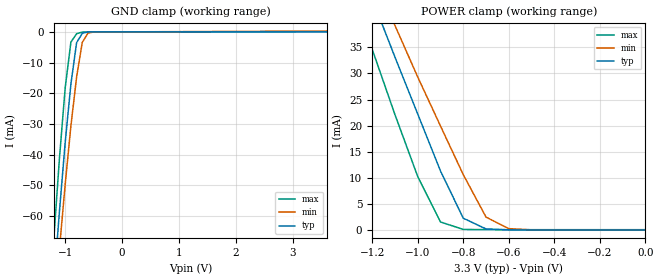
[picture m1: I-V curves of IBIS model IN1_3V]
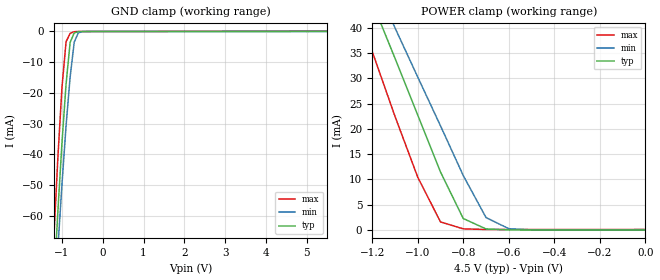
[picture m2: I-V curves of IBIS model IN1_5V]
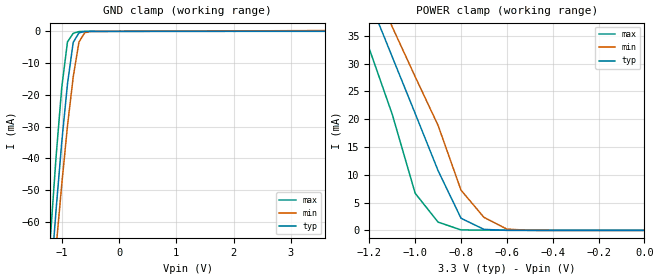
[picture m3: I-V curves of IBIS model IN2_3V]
[IBIS Ver]   5.0
[File Name]   1273na084.ibs
[File Rev]   1.0
[Date]   July 11, 2019
[Source]   JSC NIIET
[Disclaimer]
|   IBIS MODEL LICENSE AND DISCLAIMER AGREEMENT
|  Before downloading or using the below-referenced IBIS model, please read and
|  accept the license agreement and disclaimer shown below.
|   LICENSE STATEMENT
|  The information in this IBIS model is protected under the copyright laws of
|  the Russia and other countries. JSC NIIET hereby
|  grants the users of this IBIS model (hereto referred to as licensee) a
|  nonexclusive, nontransferable license to use this IBIS model as long as the
|  licensee abides by the terms of this agreement.
|  Before using the IBIS model, the licensee should read this license. By using,
|  copying, modifying or redistributing this IBIS model,licensee accepts and
|  agrees to become bound by the terms of this agreement. If the licensee does
|  not accept these terms, then the licensee should not use the IBIS model and
|  should return it to JSC NIIET immediately.
|  The licensee may not sell, loan, rent, lease, distribute or license the IBIS
|  model,in whole, in part, or in modified form, to anyone outside the
|  licensee's company. The licensee may modify the IBIS model to suit his
|  specific applications, provided that all rights in such modifications and
|  derivative works shall belong to JSC NIIET. The licensee may make copies of this
|  IBIS model for use within his company only.
|  THIS IBIS MODEL IS PROVIDED AS IS, WHERE IS, AND WITH NO WARRANTY OF ANY
|  KIND EITHER EXPRESSED OR IMPLIED, INCLUDING BUT NOT LIMITED TO ANY IMPLIED
|  WARRANTIES OF MERCHANTABILITY AND FITNESS FOR A PARTICULAR PURPOSE.
|  Licensee understands that the mathematical behavioral characteristics and
|  formulas for the IBIS model have not been fully characterized for production
|  specification or exact compliance to actual part operation. The IBIS model
|  is useful for general simulations but not intended for safety critical,
|  manufacturing yield, or similar safety or financial decision making
|  simulations. In no event will JSC NIIET be liable for indirect, special,
|  collateral, incidental, consequential or punitive damages in connection with
|  or arising out of the use of this IBIS model. JSC NIIET reserves the right to
|  make changes to its products and the IBIS model without prior notice.
|  The Parties agree that the foregoing terms constitute the entire agreement
|  and that this agreement shall be governed by and construed in accordance
|  with the laws of the Russsia, without regard to choice of law provisions.
[Copyright]
|  This model is an exclusive property of JSC NIIET
|  and is not to be resold or redistributed without the written
|  permission of JSC NIIET.
|  Copyright(c) 2019 JSC NIIET, All Rights Reserved
|   Component 1273HA084
[Component]   1273HA084
[Manufacturer] JSC NIIET
[Package]
| variable   typ   min   max
R_pkg   0   NA   NA
L_pkg   0   NA   NA
C_pkg   0   NA   NA
[Pin]   signal_name   model_name   R_pin   L_pin   C_pin
1   NC   NC   NA   NA   NA
2   #VCC   POWER   NA   NA   NA
3   NC   NC   NA   NA   NA
4   MOSI/ADR1   IN1   NA   NA   NA
5   MISO/SDA   IO   NA   NA   NA
6   SCLK/SCL   IN1   NA   NA   NA
7   SS#/ADR0   IN1   NA   NA   NA
8   SA_MODE   IN1   NA   NA   NA
9   PU/RST#   IN2   NA   NA   NA
10   NC   NC   NA   NA   NA
11   AGND   GND   NA   NA   NA
12   VCC1   POWER   NA   NA   NA
13   DAC1P   TERM   NA   NA   NA
14   DAC1N   TERM   NA   NA   NA
15   DAC2P   TERM   NA   NA   NA
16   DAC2N   TERM   NA   NA   NA
17   DAC3P   TERM   NA   NA   NA
18   DAC3N   TERM   NA   NA   NA
19   DAC4P   TERM   NA   NA   NA
20   DAC4N   TERM   NA   NA   NA
21   VCC2   POWER   NA   NA   NA
22   DAC_BIAS1   TERM   NA   NA   NA
23   DAC_BIAS2   TERM   NA   NA   NA
24   AGND   GND   NA   NA   NA
25   CM   TERM   NA   NA   NA
26   TS_REF   TERM   NA   NA   NA
27   DAC5P   TERM   NA   NA   NA
28   DAC5N   TERM   NA   NA   NA
29   DAC6P   TERM   NA   NA   NA
30   DAC6N   TERM   NA   NA   NA
31   DAC7P   TERM   NA   NA   NA
32   DAC7N   TERM   NA   NA   NA
33   DAC8P   TERM   NA   NA   NA
34   DAC8N   TERM   NA   NA   NA
35   DAC9P   TERM   NA   NA   NA
36   DAC9N   TERM   NA   NA   NA
37   DAC10P   TERM   NA   NA   NA
38   DAC10N   TERM   NA   NA   NA
39   DAC11P   TERM   NA   NA   NA
40   DAC11N   TERM   NA   NA   NA
41   DAC12P   TERM   NA   NA   NA
42   DAC12N   TERM   NA   NA   NA
43   AGND   GND   NA   NA   NA
44   DAC_BIAS3   TERM   NA   NA   NA
45   DAC_BIAS4   TERM   NA   NA   NA
46   VCC3   POWER   NA   NA   NA
47   VCC3   POWER   NA   NA   NA
48   DAC13P   TERM   NA   NA   NA
49   DAC13N   TERM   NA   NA   NA
50   DAC14P   TERM   NA   NA   NA
51   DAC14N   TERM   NA   NA   NA
52   DAC15P   TERM   NA   NA   NA
53   SUBS   TERM   NA   NA   NA
54   DAC15N   TERM   NA   NA   NA
55   VCC4   POWER   NA   NA   NA
56   AGND   GND   NA   NA   NA
57   SUBS   TERM   NA   NA   NA
58   DAC16P   TERM   NA   NA   NA
59   DAC16N   TERM   NA   NA   NA
60   PLLGND   GND   NA   NA   NA
61   LF   TERM   NA   NA   NA
62   PLLVCC   POWER   NA   NA   NA
63   MCLKI/XT1   TERM   NA   NA   NA
64   XTALO   TERM   NA   NA   NA
65   MCLKO   TERM   NA   NA   NA
66   #VCC   POWER   NA   NA   NA
67   NC   NC   NA   NA   NA
68   #GND   GND   NA   NA   NA
69   NC   NC   NA   NA   NA
70   IOVCC   POWER   NA   NA   NA
71   VSENSE   TERM   NA   NA   NA
72   VDRIVE   TERM   NA   NA   NA
73   VSUPPLY   TERM   NA   NA   NA
74   #GND   GND   NA   NA   NA
75   DBCLK   IO   NA   NA   NA
76   DLRCLK   IO   NA   NA   NA
77   #VCC   POWER   NA   NA   NA
78   #GND   GND   NA   NA   NA
79   DSDATA8   IN1   NA   NA   NA
80   DSDATA7   IN1   NA   NA   NA
81   DSDATA6   IN1   NA   NA   NA
82   DSDATA5   IN1   NA   NA   NA
83   DSDATA4   IN1   NA   NA   NA
84   DSDATA3   IN1   NA   NA   NA
85   DSDATA2   IN1   NA   NA   NA
86   DSDATA1   IN1   NA   NA   NA
87   IOVCC   POWER   NA   NA   NA
88   #GND   GND   NA   NA   NA
[Model selector]  IN1
IN1_3V   input pin,iovdd=3.3v
IN1_5V   input pin,iovdd=5.0v
[Model selector]  IN2
IN2_3V   input pin,iovdd=3.3v
IN2_5V   input pin,iovdd=5.0v
[Model selector]  IO
IO_3V   input/output pin,iovdd=3.3v
IO_5V   input/output pin,iovdd=5.0v
[Model]   TERM
Model_type Terminator
Polarity   Non-Inverting
C_comp   1.984800pF   1.899400pF   2.077500pF
[Temperature Range]   25   -60   85
[Voltage Range]   3.00V   2.70V   3.30V
[POWER Clamp Reference]   3.00V   2.70V   3.30V
[GND Clamp Reference]   0.00V   0.00V   0.00V
| Models and submodels in the file (7): IN1_3V (Input), IN1_5V (Input), IN2_3V (Input), IN2_5V (Input), IO_3V (I/O), IO_5V (I/O), TERM (Terminator)
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[Model]   IN1_3V
Model_type Input
Polarity   Non-Inverting
Vinl =   0.80V
Vinh =   2.10V
C_comp   1.984800pF   1.899400pF   2.077500pF
[Temperature Range]   25   -60   85
[Voltage Range]   3.30V   3.00V   3.60V
[POWER Clamp Reference]   3.30V   3.00V   3.60V
[GND Clamp Reference]   0.00V   0.00V   0.00V
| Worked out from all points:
|   GND clamp passes 1 mA (typ) near -0.72 V on its own axis
|   POWER clamp passes 1 mA (typ) near -0.74 V on its own axis
[Power Clamp]
| Voltage   I(typ)   I(min)   I(max)
-3.6V     484mA      432.6mA    558.1mA
-1.3V     56.33mA    62.02mA    47.32mA
-1.2V     44.35mA    50.06mA    34.66mA
-1.1V     33.15mA    39.21mA    22.12mA
-1V       22.24mA    29.33mA    10.25mA
-900mV    11.32mA    19.94mA    1.536mA
-800mV    2.254mA    10.61mA    102.9uA
-700mV    201.6uA    2.466mA    60.78uA
-600mV    17.58uA    255.9uA    56.81uA
-500mV    3.141uA    22.76uA    55.31uA
0V        2.597uA    1.568uA    53.5uA
[GND Clamp]
| Voltage   I(typ)   I(min)   I(max)
-3.6V     -860.2mA   -772.2mA   -995.6mA
-1.2V     -82.4mA    -92.53mA   -67.37mA
-1.1V     -58.29mA   -70.52mA   -40.93mA
-1V       -36.02mA   -49.7mA    -18.19mA
-900mV    -17.02mA   -30.67mA   -3.357mA
-800mV    -3.529mA   -14.75mA   -618.5uA
-700mV    -476.4uA   -3.425mA   -68.3uA
-600mV    -48.03uA   -439.4uA   -17.72uA
-500mV    -5.222uA   -40.96uA   -13.46uA
3.6V      0A         254.9uA    61.44uA
[Model]   IN1_5V
Model_type Input
Polarity   Non-Inverting
Vinl =   0.80V
Vinh =   2.10V
C_comp   1.984800pF   1.899400pF   2.077500pF
[Temperature Range]   25   -60   85
[Voltage Range]   4.50V   5.00V   5.50V
[POWER Clamp Reference]   4.50V   5.00V   5.50V
[GND Clamp Reference]   0.00V   0.00V   0.00V
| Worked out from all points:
|   GND clamp passes 1 mA (typ) near -0.72 V on its own axis
|   POWER clamp passes 1 mA (typ) near -0.74 V on its own axis
[Power Clamp]
| Voltage   I(typ)   I(min)   I(max)
-5.5V     814.2mA    717.5mA    973.1mA
-1.3V     56.59mA    61.7mA     48.14mA
-1.2V     45.11mA    50.36mA    35.34mA
-1.1V     33.99mA    40.01mA    22.51mA
-1V       22.76mA    30.27mA    10.46mA
-900mV    11.48mA    20.61mA    1.598mA
-800mV    2.269mA    10.77mA    223.8uA
-700mV    205.6uA    2.458mA    100.2uA
-600mV    21.67uA    254.1uA    97.93uA
-500mV    8.042uA    24.59uA    97.2uA
0V        7.553uA    4.49uA     111.6uA
[GND Clamp]
| Voltage   I(typ)   I(min)   I(max)
-5.5V     -1.461A    -1.286A    -1.729A
-1.2V     -82.64mA   -92.41mA   -67.31mA
-1.1V     -58.5mA    -70.47mA   -40.88mA
-1V       -36.18mA   -49.72mA   -18.16mA
-900mV    -17.14mA   -30.73mA   -3.343mA
-800mV    -3.559mA   -14.83mA   -610.5uA
-700mV    -479.5uA   -3.458mA   -62.83uA
-600mV    -48.82uA   -444.4uA   -8.614uA
-500mV    -6.024uA   -41.83uA   -4.63uA
5.5V      7.517uA    7.623uA    137.4uA
[Model]   IN2_3V
Model_type Input
Polarity   Non-Inverting
Vinl =   0.80V
Vinh =   2.10V
C_comp   1.984800pF   1.899400pF   2.077500pF
[Temperature Range]   25   -60   85
[Voltage Range]   3.30V   3.00V   3.60V
[POWER Clamp Reference]   3.30V   3.00V   3.60V
[GND Clamp Reference]   0.00V   0.00V   0.00V
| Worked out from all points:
|   GND clamp passes 1 mA (typ) near -0.72 V on its own axis
|   POWER clamp passes 1 mA (typ) near -0.74 V on its own axis
[Power Clamp]
| Voltage   I(typ)   I(min)   I(max)
-3.6V     396mA      354.6mA    462.2mA
-1.3V     52.01mA    56.39mA    44.38mA
-1.2V     41.41mA    46.14mA    32.65mA
-1.1V     31.21mA    36.61mA    20.88mA
-1V       21.04mA    27.65mA    6.686mA
-900mV    10.75mA    18.89mA    1.502mA
-800mV    2.203mA    7.246mA    103.7uA
-700mV    201.6uA    2.366mA    62.36uA
-600mV    17.62uA    249uA      58.7uA
-500mV    3.27uA     22.2uA     57.4uA
0V        2.734uA    1.662uA    56.8uA
[GND Clamp]
| Voltage   I(typ)   I(min)   I(max)
-3.6V     -835mA     -749.2mA   -963.5mA
-1.2V     -79.88mA   -89.79mA   -65.49mA
-1.1V     -56.51mA   -68.43mA   -39.8mA
-1V       -34.94mA   -48.25mA   -17.72mA
-900mV    -16.57mA   -29.82mA   -3.31mA
-800mV    -3.489mA   -14.41mA   -613.6uA
-700mV    -475.1uA   -3.405mA   -68.05uA
-600mV    -48.27uA   -441.5uA   -17.36uA
-500mV    -5.375uA   -41.43uA   -12.64uA
3.6V      2.714uA    254.7uA    63.53uA
